ORGANIZATION_BLOCK MAIN:OB1
TITLE=Ciclo A+/A-/B+/B-/C+/C-/D+/D-
//Simulatore: 07
//Versione: 1.0
//Data: 28/02/2002
//------------- DESCRIZIONE DEL CONTROLLO ---------------------
// L'esempio utilizza quattro cilindri (A, B, C, D) a doppio effetto
// e quattro elettrovalvole 5/2 bistabili (1V1, 2V1, 3V1, 4V1).
// Una valvola 3/2 monostabile 0V permette la distribuzione dell'aria al
// circuito.
// Se interviene un circuito di sicurezza esterno (simulato dal
// pulsante SB5) il PLC provvede ad azzerare l'uscita del distributore
// dell'aria (valvola 0V).
// Un Pulsante SB1 da inizio al ciclo ripetitivo che può essere
// interrotto dal pulsante di Stop SB3(il ciclo viene sempre terminato).
// Il pulsante SB2 da invece inizio ad un solo ciclo completo.
// Due lampade HL1, HL2 e HL3 indicano rispettivamente: la presenza
// dell'aria, il modo di funzionamento con ciclo ripetitivo e
// l'intervento del circuito di sicurezza esterna.
// I collegamenti agli ingressi del PLC sono:
// - Il selettore SA per il comando dell'aria compressa;
// - Il pulsante di arresto ciclo SB3;
// - Il pulsante di avvio ciclo in semiautomatico SB2;
// - il pulsante di avvio ciclo automatico SB1;
// - i fine corsa magnetici per il controllo della posizione
//   dei pistoni dei tre cilindri;
// - il contatto di consenso del circuito di sicurezza (simulato dal
//   pulsante SB5).
//

BEGIN
NETWORK 1 //Imposta a 1 al primo ciclo il Merker M1.3
//
LD SM0.1
S M1.3 1

NETWORK 2 //On/Off distributrice aria
//
LD I1.4
A I1.5
= Q1.0

NETWORK 3 //Imposta condizioni Start/Stop Ciclo
//
LD I1.0
O M0.0
A I1.2
= M0.0

NETWORK 4 //Corsa A+
//
LD M0.0
O I1.1
AN M1.0
A M1.3
A I0.6
= Q0.0
R M1.0 4

NETWORK 5 //Corsa A-
//
LD I0.1
= Q0.1
S M1.0 1

NETWORK 6 //Corsa B+
//
LD M1.0
AN M1.1
A I0.0
= Q0.2

NETWORK 7 //Corsa B-
//
LD I0.3
= Q0.3
S M1.1 1

NETWORK 8 //Corsa  C+
//
LDN M1.2
A M1.1
A I0.2
= Q0.4

NETWORK 9 //Corsa  C-
//
LD I0.5
= Q0.5
S M1.2 1

NETWORK 10 //Corsa D+
//
LD M1.2
AN M1.3
A I0.4
= Q0.6

NETWORK 11 //Corsa D-
//
LD I0.7
= Q0.7
S M1.3 1
R M1.0 3

NETWORK 12 //Segnalazione presenza aria
//
LD Q1.0
= Q1.1

NETWORK 13 //Segnalazione Ciclo attivo
//
LD M0.0
= Q1.2

NETWORK 14 //Segnalazione intervento emergenza esterna
//
LDN I1.4
= Q1.3

END_ORGANIZATION_BLOCK

